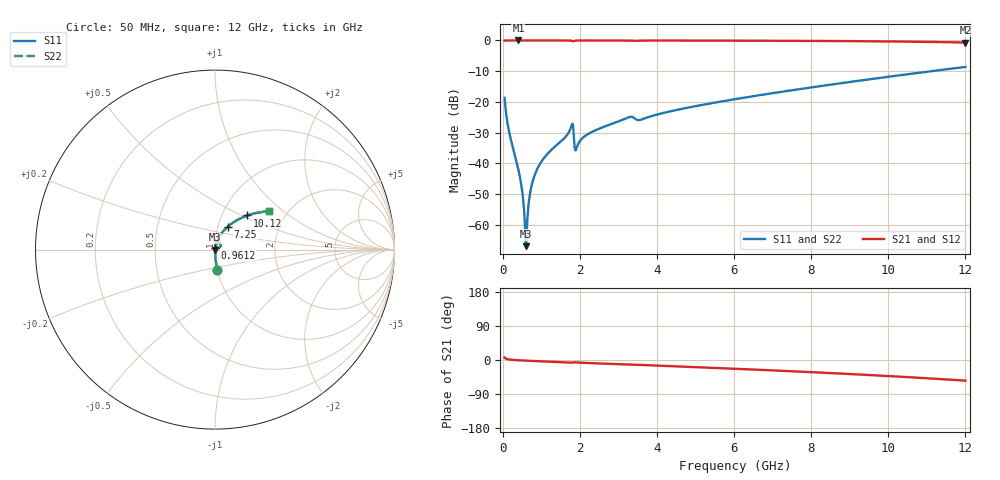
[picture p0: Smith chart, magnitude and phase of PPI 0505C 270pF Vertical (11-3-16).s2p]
# GHz S MA R 50
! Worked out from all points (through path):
!   1601 points, 50 MHz to 12 GHz, reference 50 ohm
!   highest |S21| = 0.00 dB at 408.5 MHz (marker M1); lowest = -0.7 dB at 12 GHz (marker M2)
!   group delay of S21, straight-line fit = 12.4 ps
!   lowest |S11| = -67.0 dB at 602.7 MHz (marker M3), VSWR 1.00, Z = 50 - j0.00446 ohm
!   |S11| at or under -10 dB: start of sweep to 11.12 GHz
!   |S22| runs from -67.0 to -8.6 dB; largest |S21 - S12| = 0
!   S11 on the Smith chart (normalised r, x): 50 MHz: 1.00, -0.23; 961.2 MHz: 1.00, +0.02; 7.25 GHz: 1.11, +0.29; 10.12 GHz: 1.32, +0.54; 12 GHz: 1.63, +0.80
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0.05  0.1162 -83.4  0.993 6.5  0.993 6.5  0.1162 -83.4
0.1769688  0.03041 -88.2  0.9992 1.2  0.9992 1.2  0.03041 -88.2
0.4085  0.007848 -87.9  0.9996 -0.7  0.9996 -0.7  0.007848 -87.9
0.498125  0.003813 -84.9  0.9995 -1.2  0.9995 -1.2  0.003813 -84.9
0.5653438  0.001361 -72.8  0.9995 -1.5  0.9995 -1.5  0.001361 -72.8
0.6026875  0.000449 -5.7  0.9995 -1.7  0.9995 -1.7  0.000449 -5.7
0.6400313  0.00124 66.4  0.9995 -1.9  0.9995 -1.9  0.00124 66.4
0.6997813  0.002963 78.6  0.9995 -2.1  0.9995 -2.1  0.002963 78.6
0.7595312  0.004606 81.5  0.9994 -2.4  0.9994 -2.4  0.004606 81.5
0.9611875  0.009639 83.5  0.9993 -3.3  0.9993 -3.3  0.009639 83.5
1.767813  0.03832 71.0  0.9913 -7.1  0.9913 -7.1  0.03832 71.0
1.909719  0.01731 64.9  0.9942 -6.3  0.9942 -6.3  0.01731 64.9
2.044156  0.02486 79.0  0.9979 -7.2  0.9979 -7.2  0.02486 79.0
3.261563  0.05585 72.3  0.993 -12.3  0.993 -12.3  0.05585 72.3
3.545375  0.05061 69.2  0.9915 -12.8  0.9915 -12.8  0.05061 69.2
4.038312  0.06306 73.5  0.996 -14.9  0.996 -14.9  0.06306 73.5
6.025  0.1108 66.1  0.992 -23.1  0.992 -23.1  0.1108 66.1
7.249875  0.1465 60.8  0.9871 -28.5  0.9871 -28.5  0.1465 60.8
8.019156  0.1726 57.3  0.9827 -32.1  0.9827 -32.1  0.1726 57.3
10.01331  0.2569 47.1  0.9635 -42.4  0.9635 -42.4  0.2569 47.1
10.11787  0.2621 46.5  0.9621 -43.0  0.9621 -43.0  0.2621 46.5
12  0.3707 35.1  0.925 -54.5  0.925 -54.5  0.3707 35.1
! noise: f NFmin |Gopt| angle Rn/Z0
0.05  0.0003175  0.8363  0.2478  0.0004101
1.372  0.003187  0.6084  3.713  0.001505
2.701  0.005644  0.5744  7.198  0.002395
4.031  0.008738  0.5875  10.74  0.003839
5.36  0.009006  0.4994  13.58  0.003067
6.682  0.01064  0.4808  16.45  0.00343
8.012  0.01256  0.4775  19.27  0.003989
9.341  0.01476  0.4839  22.03  0.004731
10.67  0.01735  0.4985  24.77  0.005724
12  0.02045  0.5207  27.55  0.007091
